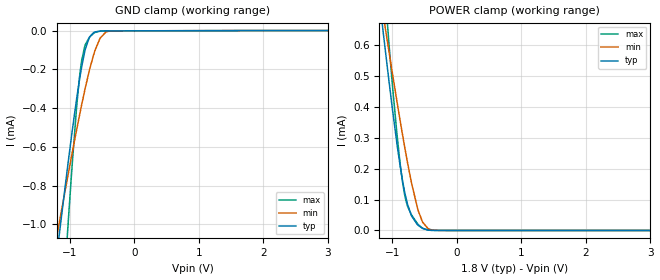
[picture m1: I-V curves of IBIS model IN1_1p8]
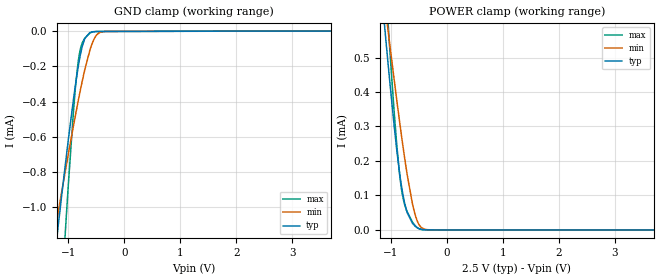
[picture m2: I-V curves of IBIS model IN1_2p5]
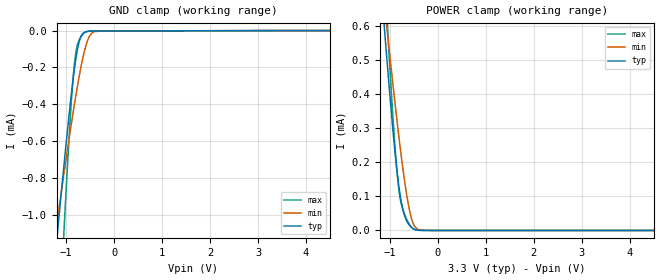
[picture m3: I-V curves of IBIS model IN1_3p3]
|Texas Instruments Incorporated
|ISO1450
[IBIS Ver]   4.1
[File name]   iso1450.ibs
[Date]   24/03/2019
[File Rev]   1.0
[Source]
| Texas Instruments Incorporated.
| Analog-eLab Design Center, HPA
| 12500 TI Blvd
| Dallas, TX -75243
[Notes]   Revision History:
| Rev 1.0: 24/03/2019
| - Initial version of the model
| - Model generated from simulations in SPECTRE
| - Model names with a trailing _1p8 contain the model for 1.8V operation.
|   Model names with a trailing _2p5 contain the model for 2.5V operation.
|   Model names with a trailing _3p3 contain the model for 3.3V operation.
|   Model names with a trailing _5p0 contain the model for 5.0V operation.
| - C_comp although listed in numerical order of value are
|   obtained from varying PVT conditions. For PVT conditions for
|   each specific value refer the buffer description under
|   respective [Model]. IBIS model user is responsible for using
|   appropriate C_comp to simulate for Signal Integrity.
[Disclaimer]
| This model is designed as an aid for customers of Texas Instruments.
| TI and its licensors and suppliers make no warranties, either expressed
| or implied, with respect to this  model, including the warranties of
| merchantability or fitness for a particular purpose. The model is
| provided solely on an "as is" basis. The entire risk as to its quality
| and performance is with the customer.
| This model is subject to change without notice. Texas Instruments
| Incorporated is not responsible for updating this model.
[Copyright]
(C) Copyright 2019 Texas Instruments Incorporated.All rights reserved.
|  Component ISO1450DW 16-Pin SOIC -DW package
|  Part # ISO1450DW
[Component]   ISO1450DW
[Manufacturer]   TI
[Package]   |16 SOIC -DW package
|   typ   min   max
R_pkg   0.05   0.04   0.06
L_pkg   1.0nH   0.8nH   1.2nH
C_pkg   0.2pF   0.16pF   0.24pF
[Pin] signal_name  model_name   R_pin   L_pin   C_pin
1   VCC1   POWER   NA   NA   NA
2   GND1   GND   NA   NA   NA
3   R   OUT   NA   NA   NA
4   REB   IN1   NA   NA   NA
5   DE   IN2   NA   NA   NA
6   D   IN1   NA   NA   NA
7   NC   NC   NA   NA   NA
8   GND1   GND   NA   NA   NA
9   GND2   GND   NA   NA   NA
10   NC   NC   NA   NA   NA
11   NC   NC   NA   NA   NA
12   A   DIFFOY   NA   NA   NA
13   B   DIFFOZ   NA   NA   NA
14   NC   NC   NA   NA   NA
15   GND2   GND   NA   NA   NA
16   VCC2   POWER   NA   NA   NA
[Diff Pin]  inv_pin  vdiff  tdelay_typ tdelay_min tdelay_max
12   13   NA   NA   NA   NA
|  Component ISO1450BDW 16-Pin SOIC -DW package
|  Part # ISO1450BDW
[Component]   ISO1450BDW
[Manufacturer]   TI
[Package]   |16 SOIC -DW package
|   typ   min   max
R_pkg   0.05   0.04   0.06
L_pkg   1.0nH   0.8nH   1.2nH
C_pkg   0.2pF   0.16pF   0.24pF
[Pin] signal_name  model_name   R_pin   L_pin   C_pin
1   VCC1   POWER   NA   NA   NA
2   GND1   GND   NA   NA   NA
3   R   OUT   NA   NA   NA
4   REB   IN1   NA   NA   NA
5   DE   IN2   NA   NA   NA
6   D   IN1   NA   NA   NA
7   NC   NC   NA   NA   NA
8   GND1   GND   NA   NA   NA
9   GND2   GND   NA   NA   NA
10   NC   NC   NA   NA   NA
11   NC   NC   NA   NA   NA
12   A   DIFFOY   NA   NA   NA
13   B   DIFFOZ   NA   NA   NA
14   NC   NC   NA   NA   NA
15   GND2   GND   NA   NA   NA
16   VCC2   POWER   NA   NA   NA
[Diff Pin]  inv_pin  vdiff  tdelay_typ tdelay_min tdelay_max
12   13   NA   NA   NA   NA
|   Model Selectors
[Model Selector] IN1
IN1_1p8   1.8V   digital Input
IN1_2p5   2.5V   digital Input
IN1_3p3   3.3V   digital Input
IN1_5p0   5.0V   digital Input
[Model Selector] IN2
IN2_1p8   1.8V   digital Input
IN2_2p5   2.5V   digital Input
IN2_3p3   3.3V   digital Input
IN2_5p0   5.0V   digital Input
[Model Selector] OUT
OUT_1p8   1.8V   digital Output
OUT_2p5   2.5V   digital Output
OUT_3p3   3.3V   digital Output
OUT_5p0   5.0V   digital Output
[Model Selector] DIFFOY
DIFFO_3p3Y   3.3V   Differential digital Output A
DIFFO_5p0Y   5.0V   Differential digital Output A
[Model Selector] DIFFOZ
DIFFO_3p3Z   3.3V   Differential digital Output B
DIFFO_5p0Z   5.0V   Differential digital Output B
| Models and submodels in the file (16): IN1_1p8 (Input), IN1_2p5 (Input), IN1_3p3 (Input), IN1_5p0 (Input), IN2_1p8 (Input), IN2_2p5 (Input), IN2_3p3 (Input), IN2_5p0 (Input), OUT_1p8 (3-state), OUT_2p5 (3-state), OUT_3p3 (3-state), OUT_5p0 (3-state), DIFFO_3p3Y (3-state), DIFFO_3p3Z (3-state), DIFFO_5p0Y (3-state), DIFFO_5p0Z (3-state)
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|   IN1_1p8 Model
[Model]   IN1_1p8
Model_type   Input
Vinl = 0.54
Vinh = 1.26
|   typ   min   max
C_comp   0.00095pF   0.00076pF   0.0142pF
|  Where Nom  PVT is Nominal Process, 1.8V,  27C
|   Fast PVT is Strong Process,  1.89V,  -40C
|   Slow PVT is Weak Process,   1.71V, 150C
[Model spec]
|subparameter
Vinl   0.54   0.513   0.567
Vinh   1.26   1.197   1.323
[Voltage Range]   1.8   1.71   1.89
|Junction Temperature
[Temperature Range]   27   150   -40
[Power Clamp Reference]   1.8   1.71   1.89
[GND Clamp Reference]   0   0   0
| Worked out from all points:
|   GND clamp passes 1 mA (typ) near -1.14 V on its own axis
|   POWER clamp passes 1 mA (typ) near -1.34 V on its own axis
[GND Clamp]
|   Voltage   I(typ)   I(min)   I(max)
-1.8V     -2.874mA   -2.195mA   -5.336mA
-1.184V   -1.11mA    -1.03mA    -1.821mA
-1.163V   -1.051mA   -990.6uA   -1.705mA
-1.028V   -686uA     -745.6uA   -1.004mA
-898.2mV  -361.3uA   -518.9uA   -411.1uA
-828mV    -209.5uA   -402uA     -181.4uA
-757.8mV  -93.79uA   -292.1uA   -71.12uA
-698.4mV  -36.2uA    -207.5uA   -35.59uA
-633.6mV  -10.97uA   -127.9uA   -14.52uA
-531mV    -2.469uA   -39.62uA   -2.975uA
-369mV    -1.445uA   -2.669uA   -1.543uA
3.6V      0A         0A         0A
[POWER Clamp]
|   Voltage   I(typ)   I(min)   I(max)
-1.8V     1.872mA    1.618mA    2.869mA
-1.179V   709.8uA    751.5uA    957.6uA
-1.055V   490uA      584.3uA    612.9uA
-919.8mV  269uA      408.1uA    296.9uA
-871.2mV  199.5uA    346.9uA    204.2uA
-817.2mV  133.9uA    281.2uA    125.6uA
-768.6mV  88.65uA    224.9uA    81.75uA
-703.8mV  48uA       155.6uA    51.14uA
-612mV    19.26uA    74.45uA    22.69uA
-531mV    6.785uA    27.03uA    7.136uA
-293.4mV  209.8nA    425.9nA    202.8nA
3.6V      0A         0A         0A
|   IN1_2p5 Model
[Model]   IN1_2p5
Model_type   Input
Vinl = 0.75
Vinh = 1.75
|   typ   min   max
C_comp   0.00095pF   0.00076pF   0.015pF
|  Where Nom  PVT is Nominal Process, 2.5V,   27C
|   Fast PVT is Strong Process,  2.75,   -340C
|   Slow PVT is Weak Process,   2.25V,  150C
[Model spec]
|subparameter
Vinl   0.75   0.675   0.825
Vinh   1.75   1.575   1.925
[Voltage Range]   2.5   2.25   2.75
|Junction Temperature
[Temperature Range]   27   150   -40
[Power Clamp Reference]   2.5   2.25   2.75
[GND Clamp Reference]   0   0   0
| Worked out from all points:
|   GND clamp passes 1 mA (typ) near -1.14 V on its own axis
[GND Clamp]
|   Voltage   I(typ)   I(min)   I(max)
-2.5V     -4.931mA   -3.55mA    -9.461mA
-1.232V   -1.244mA   -1.119mA   -2.084mA
-1.12V    -933.5uA   -912.3uA   -1.477mA
-1.038V   -711.7uA   -763uA     -1.052mA
-910mV    -389.1uA   -539.1uA   -459uA
-820mV    -194.3uA   -389.1uA   -163uA
-782.5mV  -129.3uA   -329.8uA   -97.62uA
-707.5mV  -42.82uA   -219.9uA   -40.05uA
-617.5mV  -8.649uA   -110.7uA   -11.7uA
-497.5mV  -2.387uA   -23.45uA   -2.737uA
-355mV    -1.896uA   -2.716uA   -2.116uA
5V        0A         0A         0A
[POWER Clamp]
|   Voltage   I(typ)   I(min)   I(max)
-2.5V     3.216mA    2.616mA    5.089mA
-1.113V   590.9uA    661.5uA    768.3uA
-1.067V   512uA      601.2uA    646.2uA
-1.03V    447.5uA    551.4uA    549.6uA
-902.5mV  243.4uA    386.1uA    262.1uA
-842.5mV  162.8uA    311.7uA    158.7uA
-805mV    121.3uA    266.8uA    112.2uA
-722.5mV  57.6uA     174.8uA    58.38uA
-617.5mV  20.43uA    78.61uA    24.1uA
-497.5mV  3.903uA    15.71uA    3.749uA
-257.5mV  171.2nA    276.9nA    172.3nA
5V        0A         0A         0A
|   IN1_3p3 Model
[Model]   IN1_3p3
Model_type   Input
Vinl = 0.99
Vinh = 2.31
|   typ   min   max
C_comp   0.00096pF   0.00076pF   0.016pF
|  Where Nom  PVT is Nominal Process, 3.3V,   27C
|   Fast PVT is Strong Process,  3.6V,   -40C
|   Slow PVT is Weak Process,   3.0V,   150C
[Model spec]
|subparameter
Vinl   0.99   0.9   1.08
Vinh   2.31   2.1   2.52
[Voltage Range]   3.3   3   3.6
|Junction Temperature
[Temperature Range]   27   150   -40
[Power Clamp Reference]   3.3   3   3.6
[GND Clamp Reference]   0   0   0
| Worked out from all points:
|   GND clamp passes 1 mA (typ) near -1.14 V on its own axis
|   POWER clamp passes 1 mA (typ) near -1.34 V on its own axis
[GND Clamp]
|   Voltage   I(typ)   I(min)   I(max)
-3.3V     -7.303mA   -5.115mA   -14.21mA
-1.211V   -1.185mA   -1.08mA    -1.967mA
-1.152V   -1.02mA    -970.3uA   -1.646mA
-1.112V   -912uA     -897.9uA   -1.436mA
-1.033V   -699.6uA   -754.9uA   -1.03mA
-904.2mV  -375.5uA   -529.2uA   -435.5uA
-815.1mV  -185.3uA   -381.3uA   -152.7uA
-716.1mV  -49.91uA   -231.9uA   -44.58uA
-597.3mV  -6.774uA   -90.92uA   -9.051uA
-458.7mV  -2.634uA   -12.21uA   -2.924uA
-260.7mV  -2.357uA   -2.487uA   -2.627uA
6.6V      0A         0A         0A
[POWER Clamp]
|   Voltage   I(typ)   I(min)   I(max)
-3.3V     4.765mA    3.768mA    7.646mA
-1.132V   625.4uA    687.7uA    822.6uA
-1.102V   572.7uA    647.7uA    739.9uA
-1.082V   538uA      621.1uA    686uA
-1.023V   435.6uA    542.1uA    532.2uA
-894.3mV  231.5uA    375.8uA    246.2uA
-805.2mV  121.5uA    267uA      112.4uA
-716.1mV  54.13uA    168.1uA    55.82uA
-617.1mV  20.34uA    78.3uA     23.99uA
-547.8mV  8.703uA    34.54uA    9.499uA
-468.6mV  2.306uA    9.387uA    2.038uA
6.6V      0A         0A         0A
